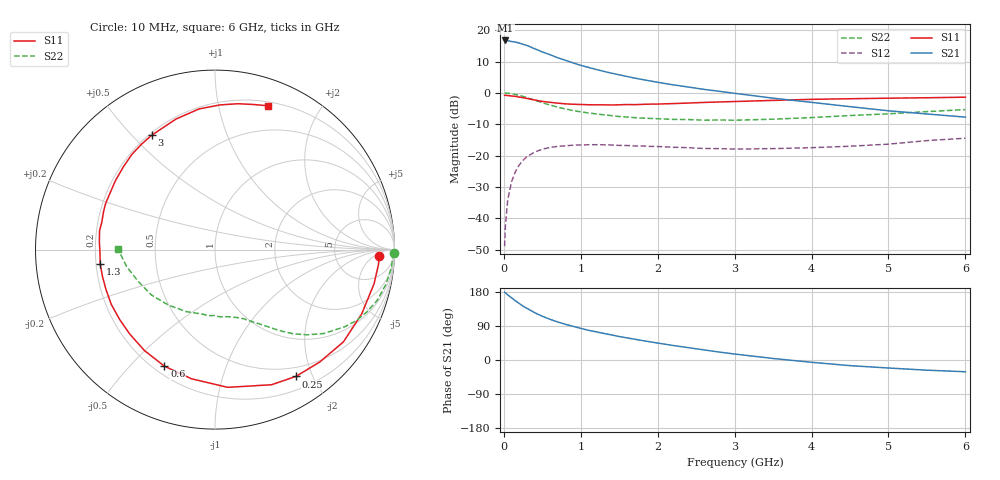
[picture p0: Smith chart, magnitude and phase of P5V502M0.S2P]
! SIEMENS Small Signal Semiconductors
! BFP183
! Si NPN RF Bipolar Junction Transistor in SOT143
! VCE = 0.5 V  IC = 2 mA
! Common Emitter S-Parameters:  March  1996
# GHz  S  MA  R  50
!  f  S11  S21  S12  S22
! GHz  MAG  ANG  MAG  ANG  MAG  ANG  MAG  ANG
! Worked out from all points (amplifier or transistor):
!   36 points, 10 MHz to 6 GHz, reference 50 ohm
!   highest |S21| = 16.7 dB at 20 MHz (marker M1)
!   |S21| within 3 dB of that: start of sweep to 435.7 MHz
!   unconditionally stable (mu >= 1): 1.927 GHz to end of sweep
!   at 250 MHz: K = 0.14, MSG = 18.5 dB, |S12| = -21.5 dB
!   at 1.4 GHz: K = 0.73, MSG = 11.4 dB, |S12| = -16.6 dB
!   at 6 GHz: K = 1.24, MAG = 0.4 dB, |S12| = -14.5 dB
!   S11 on the Smith chart (normalised r, x): 10 MHz: 18, -9; 250 MHz: 0.37, -1.76; 600 MHz: 0.24, -0.63; 1.3 GHz: 0.22, -0.06; 3 GHz: 0.21, +0.57; 6 GHz: 0.24, +1.41
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0.01  0.9146 -2.4  6.77 178.7  0.0036 86.3  0.9964 -1.1
0.02  0.9148 -5.1  6.85 177.4  0.0075 85.9  0.9909 -2.3
0.05  0.9065 -12.1  6.766 172.0  0.0196 84.0  0.988 -5.9
0.1  0.8924 -23.7  6.594 164.2  0.0381 75.7  0.9709 -11.7
0.15  0.8811 -35.7  6.454 156.4  0.0554 69.1  0.9474 -17.3
0.2  0.8561 -47.0  6.23 149.1  0.0709 63.5  0.9156 -22.2
0.25  0.8381 -57.5  5.948 142.2  0.0843 57.5  0.8796 -26.9
0.3  0.8161 -67.3  5.704 136.3  0.0962 52.5  0.839 -30.9
0.4  0.7708 -84.7  5.062 124.9  0.1139 43.6  0.7647 -37.7
0.5  0.7315 -100.3  4.489 115.4  0.1266 36.2  0.6977 -42.9
0.6  0.708 -113.5  4.07 107.4  0.1349 30.6  0.6402 -47.1
0.7  0.6861 -125.0  3.632 100.4  0.1403 25.5  0.5915 -50.4
0.8  0.6683 -135.5  3.311 94.2  0.1433 21.5  0.5536 -53.1
1.1  0.6468 -160.0  2.549 78.4  0.1488 12.6  0.4783 -59.5
1.3  0.6447 -172.9  2.2 70.1  0.1486 8.2  0.4463 -63.3
1.7  0.649 166.1  1.721 54.9  0.1428 2.9  0.4028 -70.8
2.2  0.6752 145.1  1.344 38.3  0.1361 0.0  0.3779 -81.0
3  0.7281 119.0  0.984 15.8  0.127 1.1  0.3663 -101.2
3.5  0.7589 106.7  0.823 4.0  0.1293 3.7  0.3807 -114.8
4.5  0.8067 88.0  0.603 -14.9  0.1411 8.0  0.4352 -144.4
5.5  0.8363 75.2  0.461 -26.9  0.1735 9.3  0.5028 -169.6
6  0.8537 69.8  0.411 -31.0  0.1892 6.6  0.5414 179.4
